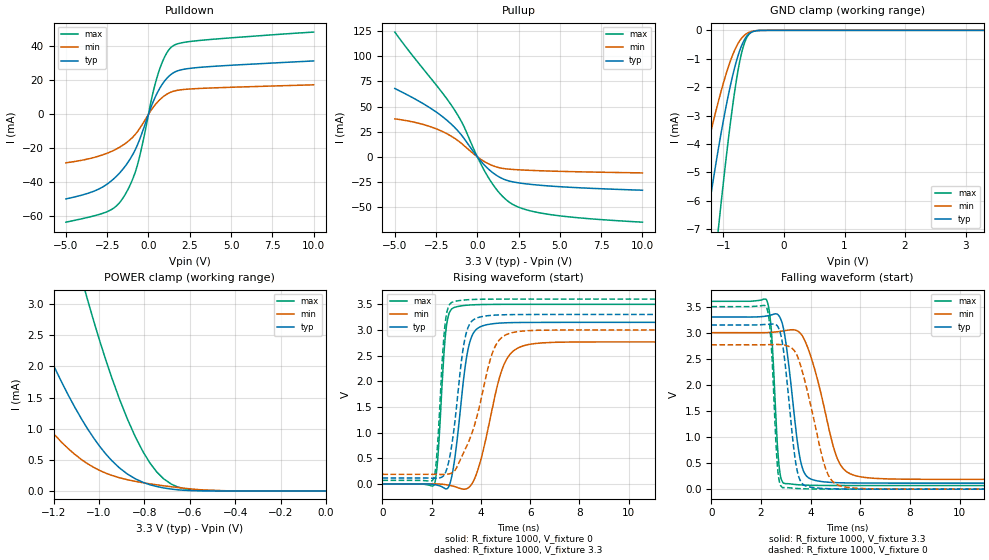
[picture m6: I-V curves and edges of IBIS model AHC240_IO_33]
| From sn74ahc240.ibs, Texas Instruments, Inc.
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[Model]   AHC240_IO_33
Model_type  3-state
Enable   Active-Low
Vref =   0
Rref =   1000
Cref =   50p
Vmeas =   1.65
| variable   typ   min   max
C_comp   2.17pF   1.98pF   2.26pF
| C_pullup   2.98pF   2.18pF   3.59pF
| C_pulldown   2.79pF   2.28pF   3.48pF
| C_tri-state   2.17pF   1.98pF   2.26pF
[Temperature Range]   40   100   -40
| Ambient temperature   25   85   -40
[Voltage range]   3.3   3   3.6
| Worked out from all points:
|   slope of the pulldown table from 0 to 0.495 V, typ, clamps not added: 41.5 ohm
|   slope of the pullup table from 0 to 0.495 V, typ, clamps not added: 52.9 ohm
|   GND clamp passes 1 mA (typ) near -0.77 V on its own axis
|   POWER clamp passes 1 mA (typ) near -1.05 V on its own axis
|   rising waveform, R_fixture 1000, V_fixture 0: 20-80 % time 461ps typ, 808ps min, 262ps max; typ from 0 V to 3.15 V
|   falling waveform, R_fixture 1000, V_fixture 3.3: 20-80 % time 470ps typ, 878ps min, 232ps max; typ from 3.3 V to 0.115 V
|   rising waveform, R_fixture 1000, V_fixture 3.3: 20-80 % time 473ps typ, 955ps min, 261ps max; typ from 0.115 V to 3.3 V
|   falling waveform, R_fixture 1000, V_fixture 0: 20-80 % time 417ps typ, 812ps min, 217ps max; typ from 3.15 V to 0 V
[GND Clamp]
| AHC240_IO_33
|   Voltage   I(typ)   I(min)   I(max)
-5V       -86.37mA   -56.48mA   -109.4mA
-1.55V    -11.02mA   -6.97mA    -17.41mA
-1.5V     -10.2mA    -6.438mA   -16.22mA
-1.295V   -7.045mA   -4.381mA   -11.51mA
-1.27V    -6.683mA   -4.145mA   -10.96mA
-1.075V   -4.064mA   -2.435mA   -6.816mA
-905mV    -2.142mA   -1.202mA   -3.604mA
-780mV    -1.044mA   -546.7uA   -1.682mA
-675mV    -421.1uA   -217.2uA   -596.1uA
-625mV    -235.4uA   -126.9uA   -301uA
-550mV    -79.25uA   -49.22uA   -83.62uA
3.3V      8.703nA    24.35nA    41.55nA
[POWER Clamp]
| AHC240_IO_33
|   Voltage   I(typ)   I(min)   I(max)
-5V       75.68mA    48.36mA    122.9mA
-1.595V   5.897mA    3.159mA    12.53mA
-1.345V   3.264mA    1.609mA    7.645mA
-1.315V   2.988mA    1.452mA    7.116mA
-1.195V   1.98mA     900.5uA    5.136mA
-1.075V   1.146mA    499uA      3.399mA
-1.05V    997.5uA    437uA      3.07mA
-945mV    493.1uA    251.9uA    1.836mA
-840mV    195.2uA    153.7uA    872uA
-715mV    48.2uA     82.85uA    194.4uA
-590mV    4.156uA    30.5uA     16.27uA
-84.45fV  8.703nA    1.32nA     64.22nA
[Pulldown]
| AHC240_IO_33
|   Voltage   I(typ)   I(min)   I(max)
-5V       -49.7mA    -28.48mA   -63.37mA
-2.43V    -40.48mA   -22.54mA   -56.87mA
-1.9V     -35.99mA   -20.13mA   -53.44mA
-1.44V    -30.85mA   -17.36mA   -47.56mA
-995mV    -24.34mA   -13.8mA    -38.95mA
-660mV    -17.77mA   -10.04mA   -29.48mA
230mV     6.092mA    3.406mA    10.92mA
590mV     13.7mA     7.69mA     24.03mA
1.015V    20.06mA    11.25mA    34.45mA
1.43V     23.93mA    13.32mA    39.88mA
2.99V     27.54mA    15.19mA    43.35mA
10V       31.4mA     17.36mA    48.36mA
[Pullup]
| AHC240_IO_33
|   Voltage   I(typ)   I(min)   I(max)
-5V       68.03mA    37.8mA     124.2mA
-3.015V   50.27mA    30.92mA    82.16mA
-2.18V    40.86mA    25.7mA     64.97mA
-1.495V   31.22mA    19.69mA    49.47mA
-870mV    19.71mA    12.08mA    32.09mA
10mV      -211.2uA   -125.8uA   -347.2uA
585mV     -10.82mA   -6.21mA    -18.35mA
1.225V    -19.11mA   -10.41mA   -33.79mA
1.86V     -23.78mA   -12.17mA   -44.23mA
2.745V    -26.46mA   -13.12mA   -51.59mA
4.22V     -28.85mA   -14.07mA   -57mA
10V       -33.24mA   -15.99mA   -65.05mA
[Ramp]
| AHC240_IO_33
| variable   typ   min   max
dV/dt_r   1.95/4.78E-10   1.72/8.39E-10   2.12/2.71E-10
dV/dt_f   1.95/4.86E-10   1.72/9.00E-10   2.14/2.46E-10
R_load = 1000
[Rising Waveform]
| AHC240_IO_33
R_fixture =   1000
C_fixture =   0
L_fixture =   0
V_fixture =   0
V_fixture_min = 0
V_fixture_max = 0
|   Time   V(typ)   V(min)   V(max)
0s        1.747nV    2.928nV    1.024nV
2.11ns    -13.29mV   721.4uV    -19.45mV
2.25ns    -27.14mV   -706uV     502mV
2.615ns   -94.44mV   -17.56mV   3.117V
2.89ns    335.7mV    -45.49mV   3.43V
3.255ns   1.858V     -100.3mV   3.471V
3.805ns   3.005V     172.9mV    3.49V
4.945ns   3.136V     2.329V     3.497V
6.16ns    3.145V     2.732V     3.498V
50ns      3.146V     2.766V     3.498V
[Falling Waveform]
| AHC240_IO_33
R_fixture =   1000
C_fixture =   0
L_fixture =   0
V_fixture =   3.3
V_fixture_min = 3
V_fixture_max = 3.6
|   Time   V(typ)   V(min)   V(max)
0s        3.3V       3V         3.6V
2.235ns   3.32V      3.001V     3.615V
2.42ns    3.34V      3.006V     3.022V
2.725ns   3.321V     3.022V     463.2mV
2.995ns   2.832V     3.041V     105.3mV
3.49ns    825.3mV    3.026V     84.78mV
3.765ns   297mV      2.846V     77.71mV
5.095ns   124mV      564.3mV    70.07mV
6.18ns    116.8mV    224.2mV    69.48mV
50ns      115.4mV    187.2mV    69.36mV
[Rising Waveform]
| AHC240_IO_33
R_fixture =   1000
C_fixture =   0
L_fixture =   0
V_fixture =   3.3
V_fixture_min = 3
V_fixture_max = 3.6
|   Time   V(typ)   V(min)   V(max)
0s        115.4mV    187.2mV    69.36mV
2.1ns     109.2mV    186.8mV    127.5mV
2.23ns    110.1mV    185.8mV    689mV
2.57ns    228.7mV    185.2mV    3.204V
3.115ns   1.983V     418.9mV    3.57V
3.345ns   2.81V      655mV      3.583V
3.62ns    3.163V     965.6mV    3.591V
4.565ns   3.287V     2.662V     3.599V
5.59ns    3.299V     2.972V     3.6V
50ns      3.3V       3V         3.6V
[Falling Waveform]
| AHC240_IO_33
R_fixture =   1000
C_fixture =   0
L_fixture =   0
V_fixture =   0
V_fixture_min = 0
V_fixture_max = 0
|   Time   V(typ)   V(min)   V(max)
0s        3.146V     2.766V     3.498V
2.22ns    3.158V     2.769V     3.493V
2.405ns   3.163V     2.772V     2.821V
2.67ns    3.121V     2.773V     398.3mV
2.88ns    2.748V     2.766V     26.71mV
3.465ns   338.8mV    2.551V     12.55mV
4.14ns    28.43mV    1.314V     3.228mV
4.78ns    7.95mV     212.1mV    1.057mV
5.87ns    1.241mV    16.48mV    186.7uV
50ns      -3.242nV   -2.615nV   -617pV
